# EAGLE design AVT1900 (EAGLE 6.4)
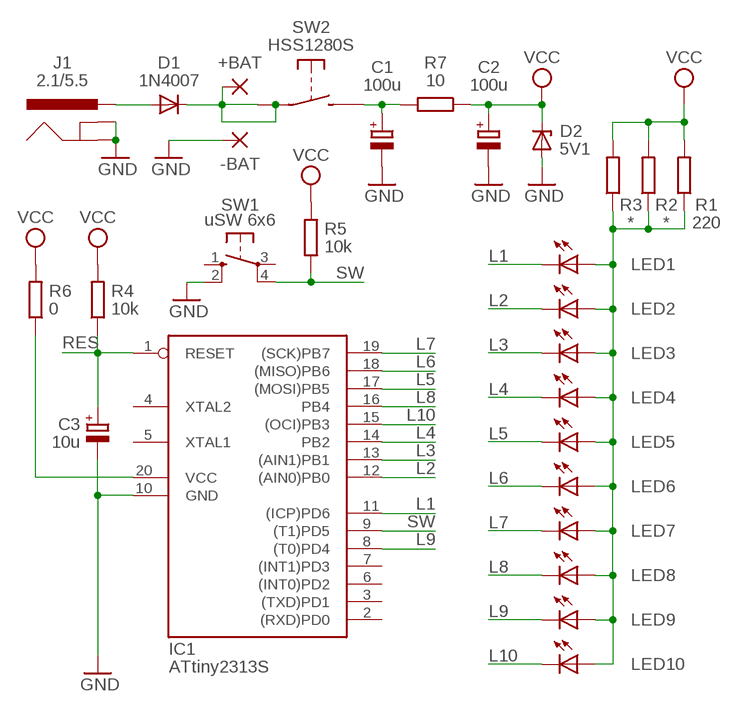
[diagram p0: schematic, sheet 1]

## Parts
+BAT  SMD5  [SMD2,54-5,08]
-BAT  SMD5  [SMD2,54-5,08]
C1  100u  CPOL-EUSMCD  [SMC_D]
C2  100u  CPOL-EUSMCD  [SMC_D]
C3  10u  CPOL-EUSMCA  [SMC_A]
D1  1N4007  DIODE-MELF-MLL41  [MELF-MLL41]
D2  5V1  ZENER-DIODESOD80C  [SOD80C]
IC1  ATtiny2313S  AT90S2313S  [SO20L]
J1  2.1/5.5  POWER_JACKSMD  [POWER_JACK_SMD]
LED1  LED3MM  [LED3MM]
LED2  LED3MM  [LED3MM]
LED3  LED3MM  [LED3MM]
LED4  LED3MM  [LED3MM]
LED5  LED3MM  [LED3MM]
LED6  LED3MM  [LED3MM]
LED7  LED3MM  [LED3MM]
LED8  LED3MM  [LED3MM]
LED9  LED3MM  [LED3MM]
LED10  LED3MM  [LED3MM]
R1  220  R-EU_R1206  [R1206]
R2  *  R-EU_R1206  [R1206]
R3  *  R-EU_R1206  [R1206]
R4  10k  R-EU_R1206  [R1206]
R5  10k  R-EU_R1206  [R1206]
R6  0  R-EU_R1206  [R1206]
R7  10  R-EU_R1206  [R1206]
SW1  uSW 6x6  10-XX_SMD  [B3F-10XX_SMD]
SW2  HSS1280S  [HSS1280S]

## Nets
GND: -BAT.1(P) C1.- C2.- C3.- D2.A IC1.10(GND) J1.GND(GNDBREAK) J1.P$4(GND) SW1.2(S1)
L1: IC1.11((ICP)PD6) LED1.K(C)
L2: IC1.12((AIN0)PB0) LED2.K(C)
L3: IC1.13((AIN1)PB1) LED3.K(C)
L4: IC1.14(PB2) LED4.K(C)
L5: IC1.17((MOSI)PB5) LED5.K(C)
L6: IC1.18((MISO)PB6) LED6.K(C)
L7: IC1.19((SCK)PB7) LED7.K(C)
L8: IC1.16(PB4) LED8.K(C)
L9: IC1.8((T0)PD4) LED9.K(C)
L10: IC1.15((OCI)PB3) LED10.K(C)
N$4: D1.A J1.VIN0(PWR)
N$7: LED1.A LED2.A LED3.A LED4.A LED5.A LED6.A LED7.A LED8.A LED9.A LED10.A R1.1 R2.1 R3.1
N$9: +BAT.1(P) D1.C SW2.2 SW2.5
N$10: IC1.20(VCC) R6.1
N$11: C1.+ R7.2 SW2.4
RES: C3.+ IC1.1(RESET) R4.1
SW: IC1.9((T1)PD5) R5.1 SW1.4(P1)
VCC: C2.+ D2.C R1.2 R2.2 R3.2 R4.2 R5.2 R6.2 R7.1
Unconnected: IC1.2((RXD)PD0) IC1.3((TXD)PD1) IC1.4(XTAL2) IC1.5(XTAL1) IC1.6((INT0)PD2) IC1.7((INT1)PD3) SW1.1(S) SW1.3(P) SW2.3

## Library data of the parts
+BAT -BAT = wirepad:SMD5: SMD PAD
C1-C3 = rcl:CPOL-EU: POLARIZED CAPACITOR, European symbol
D1 = diode:DIODE-: DIODE
D2 = diode:ZENER-DIODE: Z-Diode
IC1 = atmel:AT90S2313: MICROCONTROLLER 2 Kbytes FLASH 128 bytes SRAM 128 bytes EEPROM UART; OC_FARNELL: unknown; OC_NEWARK: unknown
J1 = SparkFun:POWER_JACK: Power Jack This is the standard 5.5mm barrel jack for power. The PTH is the most common, proven, reliable, footprint. All others are experimental. The Slot footprint only works if the mill layer is transmitted to the PCB fab house so be warned. Spark Fun Electronics SKU : PRT-00119. Mating wall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
LED1-LED10 = led:LED: LED
R1-R7 = rcl:R-EU_: RESISTOR, European symbol
SW1 = switch-omron:10-XX_SMD
SW2 = switch-misc:HSS1280S: AVT HSS1280S

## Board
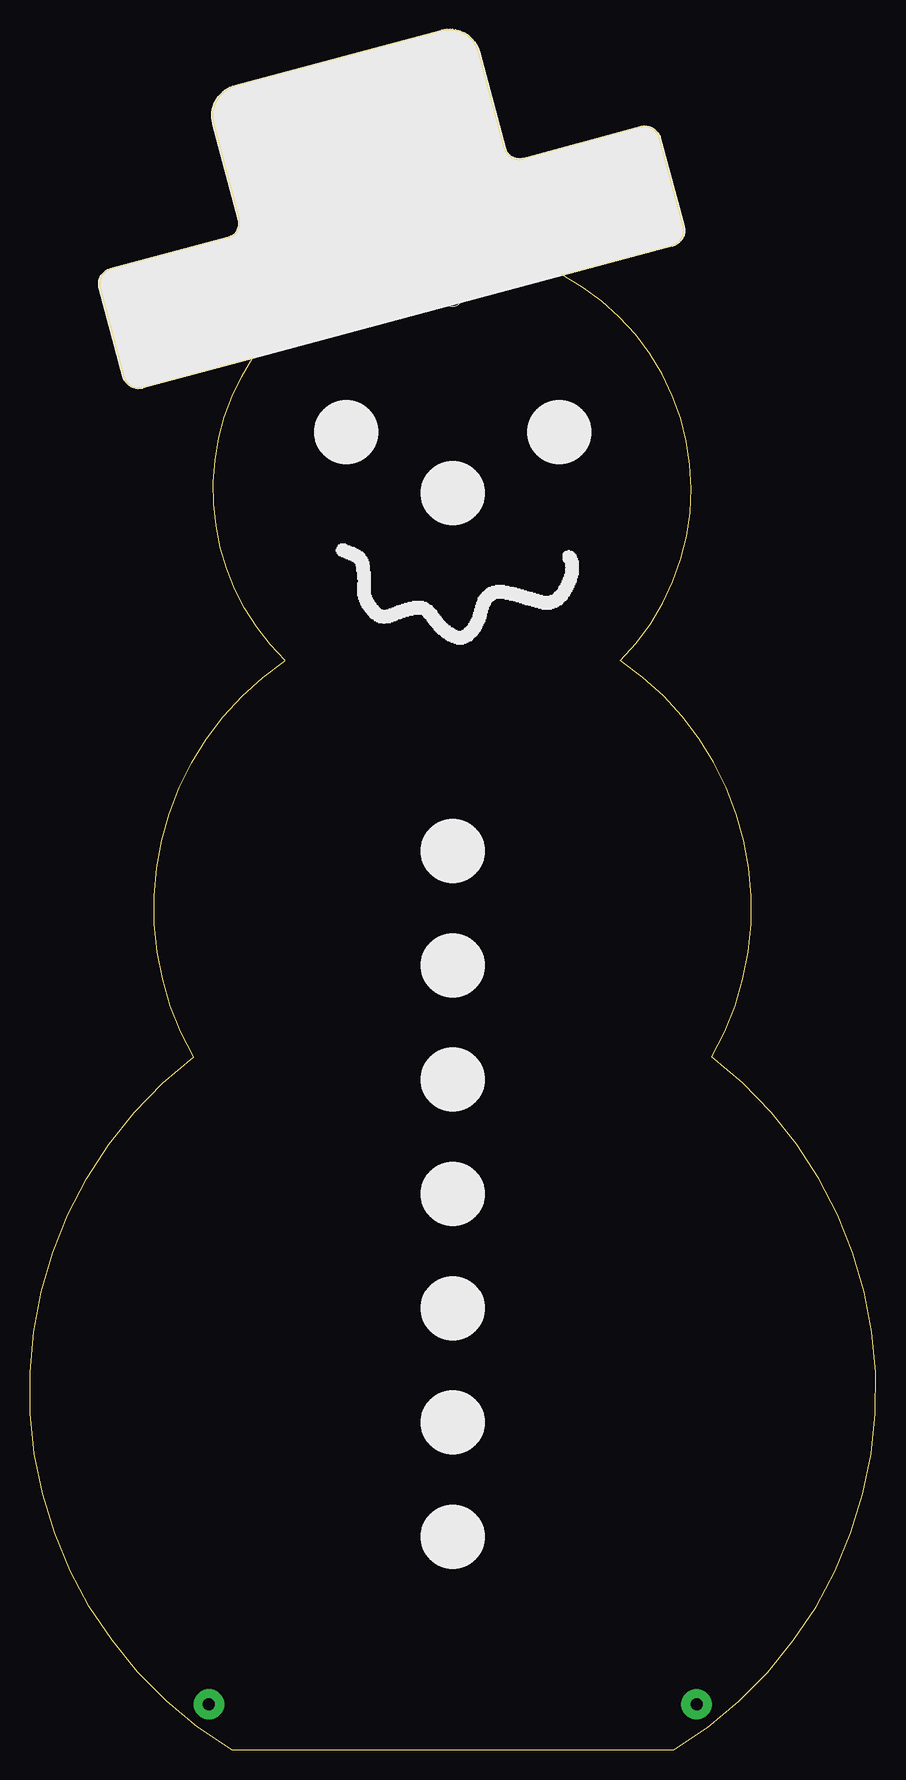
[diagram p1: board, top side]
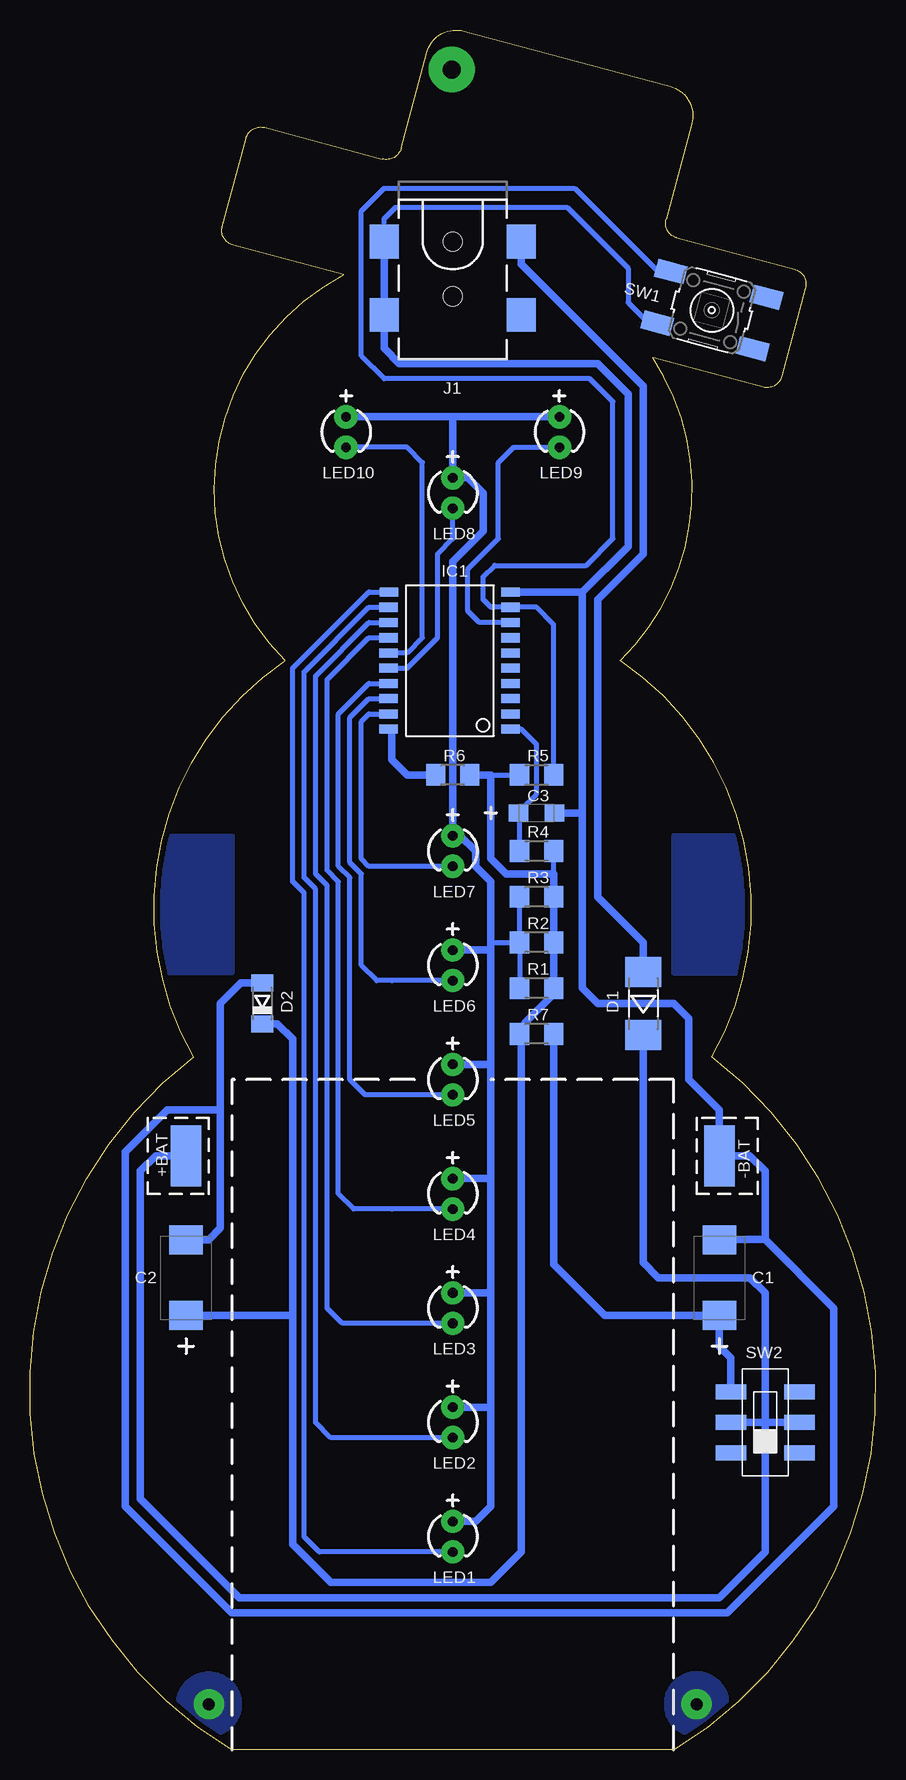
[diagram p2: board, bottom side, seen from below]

Size 70.46 x 143.37 mm. Coordinates in mm from the lower left corner, seen from the top.
Outline: 16.81,0 53.64,0 arc111 56.82,57.78 arc86 49.2,90.81 arc107 44.33,122.97 53.53,125.43 arc90 54.43,126.99 52.46,134.35 arc90 50.9,135.25 41.09,132.62 arc-90 39.53,133.52 37.4,141.49 arc90 34.28,143.29 17.11,138.68 arc90 15.31,135.57 17.45,127.6 arc-90 16.55,126.04 6.74,123.42 arc90 5.84,121.86 7.81,114.5 arc90 9.37,113.6 18.57,116.07 arc79 21.26,90.81 arc86 13.64,57.78 arc111 16.81,0
Copper layers (1*16): Top 0.035mm / dielectric 1.5mm / Bottom 0.035mm
Design rules "default *": minimum track width 10mil, minimum drill 24mil, track to track 8mil, track to pad 8mil, pad to pad 8mil, via to via 8mil, smd to smd 8mil, copper to edge 20mil, drill to drill 8mil, minimum pad ring 10mil, minimum via ring 8mil, stop-mask expansion 4mil, vias tented up to drill 0mil, thermal gap 10mil

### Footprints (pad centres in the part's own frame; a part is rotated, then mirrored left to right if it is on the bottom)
SMD2,54-5,08 = smd 2.54 x 5.08: 1 0,0
SMC_D = smd 2.4 x 2.8: + -3.15,0; - 3.15,0
SMC_A = smd 1.6 x 1.4: + -1.5,0; - 1.5,0
MELF-MLL41 = smd 2.5 x 3: A 2.625,0; C -2.625,0
SOD80C = smd 1.4 x 1.8: A 1.7,0; C -1.7,0
SO20L = smd 0.762 x 1.524: 1 -5.08,-5.448; 2 -3.81,-5.448; 3 -2.54,-5.448; 4 -1.27,-5.448; 5 0,-5.448; 6 1.27,-5.448; 7 2.54,-5.448; 8 3.81,-5.448; 9 5.08,-5.448; 10 6.35,-5.448; 11 6.35,4.686; 12 5.08,4.712; 13 3.81,4.712; 14 2.54,4.712; 15 1.27,4.712; 16 0,4.712; 17 -1.27,4.712; 18 -2.54,4.712; 19 -3.81,4.712; 20 -5.08,4.712
POWER_JACK_SMD = smd 2.8 x 2.4: GND 0,-5.7; P$4 6.1,-5.7; VIN0 0,5.7; VIN1 6.1,5.7 | hole 1.6: 0,0; 4.572,0
LED3MM = drill 0.8 pad 1.93: A -1.27,0; K 1.27,0
R1206 = smd 1.6 x 1.803: 1 -1.422,0; 2 1.422,0
B3F-10XX_SMD = smd 2.54 x 1.524: 1 -4.128,2.223; 2 4.128,2.223; 3 -4.128,-2.223; 4 4.128,-2.223
HSS1280S = smd 1.27 x 2.54: 1 6.35,-0.318; 2 8.89,-0.318; 3 11.43,-0.318; 4 11.43,5.397; 5 8.89,5.397; 6 6.35,5.397

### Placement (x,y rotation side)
+BAT  57.45,49.53 0 bottom
-BAT  13,49.53 0 bottom
C1  13,39.37 90 bottom
C2  57.45,39.37 90 bottom
C3  28.24,78.11 0 bottom
D1  19.35,62.23 90 bottom
D2  51.1,62.23 90 bottom
IC1  35.86,90.17 90 bottom
J1  35.23,125.73 270 bottom
LED1  35.23,17.78 270 bottom
LED2  35.23,27.3 270 bottom
LED3  35.23,36.83 270 bottom
LED4  35.23,46.35 270 bottom
LED5  35.23,55.88 270 bottom
LED6  35.23,65.41 270 bottom
LED7  35.23,74.93 270 bottom
LED8  35.23,104.78 270 bottom
LED9  26.34,109.86 270 bottom
LED10  44.12,109.86 270 bottom
R1  28.24,63.5 0 bottom
R2  28.24,67.31 0 bottom
R3  28.24,71.12 0 bottom
R4  28.24,74.93 0 bottom
R5  28.24,81.28 180 bottom
R6  35.23,81.28 0 bottom
R7  28.24,59.69 0 bottom
SW1  13.64,120.02 165 bottom
SW2  6.65,18.41 90 bottom

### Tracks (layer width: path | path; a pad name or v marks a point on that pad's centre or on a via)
GND
  Bottom 0.406: SW1.2 18.91,118.94 20.62,120.65 20.62,123.51 25.7,128.59 39.99,128.59 40.94,127.64 40.94,125.11 J1.GND
  Bottom 0.61: 24.43,96.52 IC1.10 | 24.43,96.52 20.62,100.33 20.62,113.03 23.16,115.57 39.67,115.57 40.94,116.84 40.94,118.98 J1.P$4 J1.GND | 24.43,78.11 C3.- | 24.43,78.11 24.43,96.52 | 24.43,78.11 24.43,63.5 23.16,62.23 16.81,62.23 15.54,60.96 15.54,55.88 13,53.34 -BAT.1 10.46,49.53 9.19,48.26 9.19,42.55 | D2.A 52.9,63.93 54.6,62.23 54.6,53.34 | 9.19,42.55 3.48,36.83 3.48,20.32 12.37,11.43 53.64,11.43 62.53,20.32 62.53,49.85 59.04,53.34 54.6,53.34 | C2.- 55.57,42.52 54.6,43.5 54.6,53.34 | 9.19,42.55 13,42.55 C1.-
GND1  (via drill 1 pad 2.54)
  other vias: 14.91,3.81
  pour Bottom: 14.83,1.27 arc-90 12.37,3.73 12.37,3.81 arc-90 14.91,6.35 arc-90 17.45,3.81 arc-90 14.91,1.27
GND2  (via drill 1 pad 2.54)
  other vias: 55.55,3.81
  pour Bottom: 55.55,1.27 arc90 58.09,3.81 arc90 55.55,6.35 arc90 53.01,3.81 arc90
L1
  Bottom 0.406: LED1.K 46.34,16.51 47.61,17.78 47.61,71.44 48.56,72.39 48.56,90.17 42.21,96.52 IC1.11
L2
  Bottom 0.406: LED2.K 45.39,26.04 46.66,27.3 46.66,71.75 47.61,72.71 47.61,89.85 42.21,95.25 IC1.12
L3
  Bottom 0.406: LED3.K 44.44,35.56 45.71,36.83 45.71,72.07 46.66,73.03 46.66,89.53 42.21,93.98 IC1.13
L4
  Bottom 0.406: LED4.K 40.31,45.09 43.48,45.09 44.75,46.35 44.75,72.39 45.71,73.34 45.71,89.22 42.21,92.71 IC1.14
L5
  Bottom 0.406: LED5.K 40.31,54.61 42.53,54.61 43.8,55.88 43.8,72.71 44.75,73.66 44.75,86.36 42.21,88.9 IC1.17
L6
  Bottom 0.406: LED6.K 40.31,64.14 41.58,64.14 42.85,65.41 42.85,73.03 43.8,73.98 43.8,86.04 42.21,87.63 IC1.18
L7
  Bottom 0.406: IC1.19 42.21,86.36 42.85,85.72 42.85,74.3 42.21,73.66 LED7.K
L8
  Bottom 0.406: IC1.16 39.04,90.17 36.5,92.71 36.5,99.69 35.23,100.97 LED8.K
L9
  Bottom 0.406: LED9.K 30.15,108.58 31.42,107.31 31.42,100.97 33.96,98.42 33.96,94.93 33.01,93.98 IC1.8
L10
  Bottom 0.406: IC1.15 39.04,91.44 37.77,92.71 37.77,107.31 39.04,108.58 LED10.K
N$2
  pour Bottom: 10.46,76.2 16.81,76.2 16.81,64.77 10.46,64.77
N$3
  pour Bottom: 53.64,64.77 59.99,64.77 59.99,76.2 53.64,76.2
N$4
  Bottom 0.61: J1.VIN0 29.53,123.84 19.35,113.67 19.35,99.69 23.16,95.89 23.16,71.12 19.35,67.31 D1.A
N$7
  Bottom 0.406: R2.1 R1.1 | R2.1 R3.1 | 32.05,67.31 R2.1
  Bottom 0.61: 32.05,47.62 32.05,57.15 | 32.05,57.15 32.05,66.67 | 32.05,57.15 LED5.A | 32.05,66.67 LED6.A | 32.05,66.67 32.05,67.31 32.05,72.39 33.32,73.66 33.32,74.93 34.59,76.2 LED7.A 35.23,99.06 32.69,101.6 32.69,104.78 33.96,106.05 LED8.A 35.23,111.12 | 32.05,47.62 LED4.A | 32.05,38.1 32.05,47.62 | 32.05,38.1 LED3.A | 32.05,28.57 LED2.A | 32.05,28.57 32.05,38.1 | LED1.A 33.32,19.05 32.05,20.32 32.05,28.57 | 35.23,111.12 LED10.A | 35.23,111.12 LED9.A
N$9
  Bottom 0.61: +BAT.1 59.99,49.53 61.26,48.26 61.26,20.95 53.01,12.7 13,12.7 9.19,16.51 9.19,27.3 | D1.C 19.35,40.64 18.08,39.37 10.46,39.37 9.19,38.1 9.19,27.3 | 9.19,27.3 SW2.2 | 9.19,27.3 SW2.5
N$10
  Bottom 0.406: 40.31,84.82 IC1.20
  Bottom 0.61: R6.1 39.04,81.28 40.31,82.55 40.31,84.82
N$11
  Bottom 0.61: R7.2 26.82,40.49 22.55,36.22 C1.+ 13,33.66 12.05,32.7 SW2.4
RES
  Bottom 0.406: IC1.1 29.51,85.09 28.24,83.82 28.24,79.69 29.51,78.42 29.51,78.33 C3.+ 29.67,78.03 R4.1
S$1  (via drill 1.5 pad 3.81)
  other vias: 35.3,140.08
SW
  Bottom 0.406: R5.1 26.82,93.83 28.24,95.25 IC1.9 32.05,95.25 32.69,95.89 32.69,97.79 31.74,98.74 24.12,98.74 21.89,100.97 21.89,112.39 23.8,114.3 40.94,114.3 42.85,116.2 42.85,128.27 40.94,130.18 25.07,130.18 18.12,123.23 SW1.4
VCC
  Bottom 0.406: 26.82,73.03 R4.2 | 26.82,63.02 R1.2 | 29.2,60.16 R7.1 29.51,59.54 | 32.05,81.28 R5.2
  Bottom 0.61: R1.2 R2.2 R3.2 26.82,73.03 30.78,73.03 32.05,74.3 32.05,81.28 R6.2 | 26.82,63.02 29.2,60.64 29.2,60.16 | 29.51,59.54 29.51,16.51 32.05,13.97 45.39,13.97 48.56,17.14 48.56,36.22 | 48.56,36.22 48.56,59.26 49.83,60.53 D2.C | 48.56,36.22 C2.+

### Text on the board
bNames: J1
